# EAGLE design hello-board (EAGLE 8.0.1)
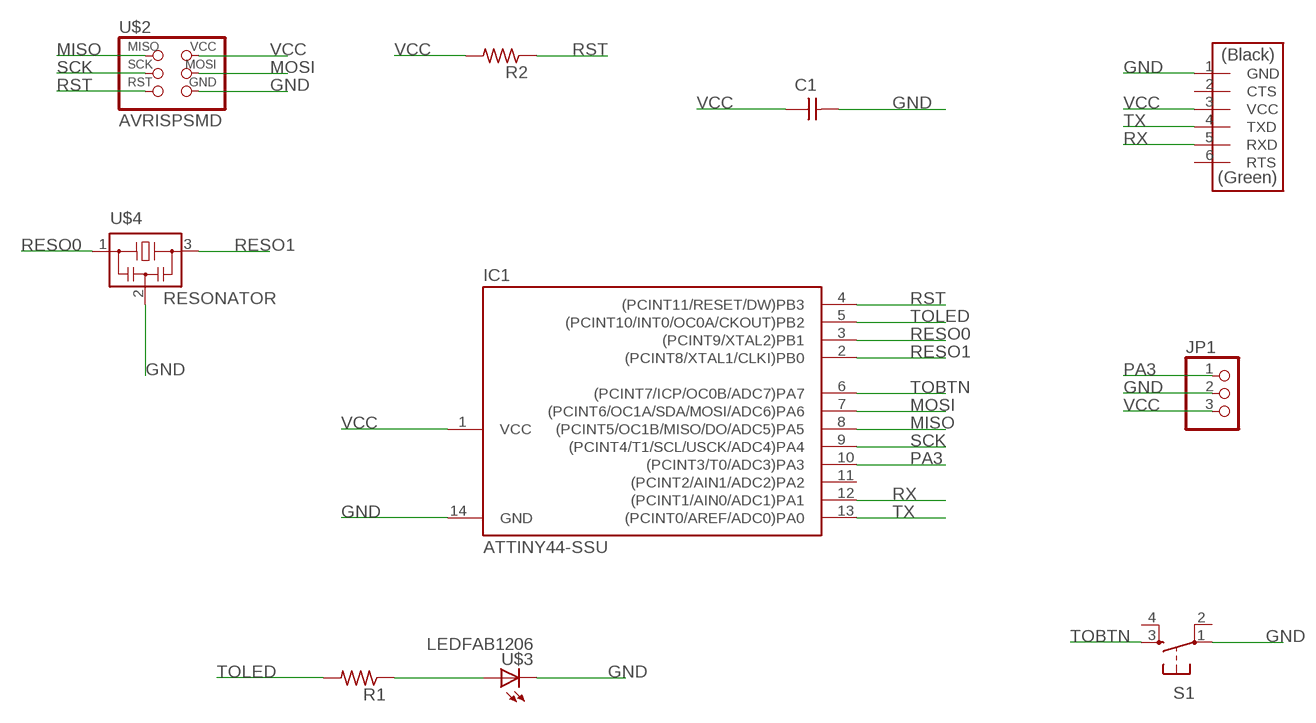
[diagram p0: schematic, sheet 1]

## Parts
C1  CAP-UNPOLARIZEDFAB  [C1206FAB]
IC1  ATTINY44-SSU  [SOIC14]
JP1  PINHD-1X3  [1X03]
R1  RES-US1206FAB  [R1206FAB]
R2  RES-US1206FAB  [R1206FAB]
S1  6MM_SWITCH6MM_SWITCH  [6MM_SWITCH]
U$1  FTDI-SMD-HEADER  [1X06SMD]
U$2  AVRISPSMD  [2X03SMD]
U$3  LEDFAB1206  [LED1206FAB]
U$4  RESONATOR  [EFOBM]

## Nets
GND: C1.2 IC1.14(GND) JP1.2 S1.1(P) U$1.1(GND) U$2.6(GND) U$3.2(C) U$4.2
MISO: IC1.8((PCINT5/OC1B/MISO/DO/ADC5)PA5) U$2.1(MISO)
MOSI: IC1.7((PCINT6/OC1A/SDA/MOSI/ADC6)PA6) U$2.4(MOSI)
N$12: R1.1 U$3.1(A)
PA3: IC1.10((PCINT3/T0/ADC3)PA3) JP1.1
RESO0: IC1.3((PCINT9/XTAL2)PB1) U$4.1
RESO1: IC1.2((PCINT8/XTAL1/CLKI)PB0) U$4.3
RST: IC1.4((PCINT11/RESET/DW)PB3) R2.1 U$2.5(RST)
RX: IC1.12((PCINT1/AIN0/ADC1)PA1) U$1.5(RXD)
SCK: IC1.9((PCINT4/T1/SCL/USCK/ADC4)PA4) U$2.3(SCK)
TOBTN: IC1.6((PCINT7/ICP/OC0B/ADC7)PA7) S1.3(S)
TOLED: IC1.5((PCINT10/INT0/OC0A/CKOUT)PB2) R1.2
TX: IC1.13((PCINT0/AREF/ADC0)PA0) U$1.4(TXD)
VCC: C1.1 IC1.1(VCC) JP1.3 R2.2 U$1.3(VCC) U$2.2(VCC)
Unconnected: IC1.11((PCINT2/AIN1/ADC2)PA2) S1.2(P1) S1.4(S1) U$1.2(CTS) U$1.6(RTS)

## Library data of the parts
C1 = 01fab:CAP-UNPOLARIZED
IC1 = 01fab:ATTINY44
JP1 = pinhead:PINHD-1X3: PIN HEADER
R1 R2 = 01fab:RES-US: Resistor (US Symbol)
S1 = 01fab:6MM_SWITCH: OMRON SWITCH
U$1 = 01fab:FTDI-SMD-HEADER
U$2 = 01fab:AVRISP
U$3 = 01fab:LED: LED
U$4 = 01fab:RESONATOR

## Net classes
0 default: width 0.406 mm, drill 0.406 mm, clearance 0.406 mm

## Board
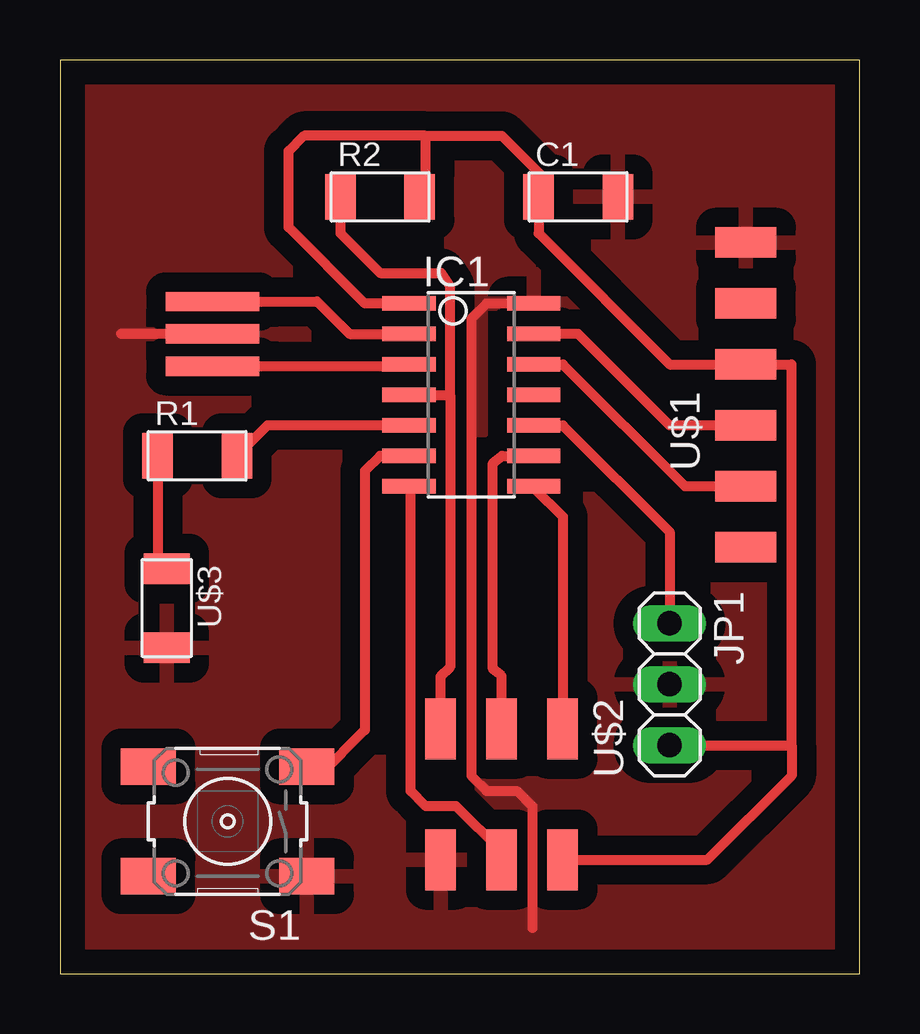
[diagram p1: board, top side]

Size 33.33 x 38.09 mm. Coordinates in mm from the lower left corner, seen from the top.
Outline: 0,0 33.33,0 33.33,38.09 0,38.09 0,0
Copper layers (1*16): Top 0.035mm / dielectric 1.5mm / Bottom 0.035mm
Design rules "default *": minimum track width 16mil, minimum drill 24mil, track to track 16mil, track to pad 16mil, pad to pad 16mil, via to via 16mil, smd to smd 16mil, copper to edge 40mil, drill to drill 8mil, minimum pad ring 10mil, minimum via ring 8mil, stop-mask expansion 4mil, vias tented up to drill 0mil, thermal gap 32mil

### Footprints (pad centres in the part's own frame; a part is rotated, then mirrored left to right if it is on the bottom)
C1206FAB = smd 1.27 x 1.905: 1 -1.651,0; 2 1.651,0
SOIC14 = smd 0.61 x 2.21: 1 -3.81,-2.603; 2 -2.54,-2.603; 3 -1.27,-2.603; 4 0,-2.603; 5 1.27,-2.603; 6 2.54,-2.603; 7 3.81,-2.603; 8 3.81,2.603; 9 2.54,2.603; 10 1.27,2.603; 11 0,2.603; 12 -1.27,2.603; 13 -2.54,2.603; 14 -3.81,2.603
1X03 = drill 1.016 long: 1 -2.54,0; 2 0,0; 3 2.54,0
R1206FAB = smd 1.27 x 1.905: 1 -1.651,0; 2 1.651,0
6MM_SWITCH = smd 2.286 x 1.524: 1 -3.302,2.286; 2 3.302,2.286; 3 -3.302,-2.286; 4 3.302,-2.286
1X06SMD = smd 2.54 x 1.27: 1 0,6.35; 2 0,3.81; 3 0,1.27; 4 0,-1.27; 5 0,-3.81; 6 0,-6.35
2X03SMD = smd 2.54 x 1.27: 1 -2.54,2.54; 2 2.92,2.54; 3 -2.54,0; 4 2.92,0; 5 -2.54,-2.54; 6 2.92,-2.54
LED1206FAB = smd 1.27 x 1.905: 1 -1.651,0; 2 1.651,0
EFOBM = smd 0.8 x 3.9: 1 -1.35,0; 2 0,0; 3 1.35,0

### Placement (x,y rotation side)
C1  21.59,32.38 0 top
IC1  17.14,24.13 270 top
JP1  25.4,12.06 270 top
R1  5.71,21.59 0 top
R2  13.34,32.38 0 top
S1  6.99,6.35 180 top
U$1  28.57,24.13 0 top
U$2  18.4,7.67 270 top
U$3  4.45,15.24 270 top
U$4  6.35,26.67 90 top

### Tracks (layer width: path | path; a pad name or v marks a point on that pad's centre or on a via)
GND
  Top 0.406: U$4.2 2.54,26.67 | 19.68,1.91 19.68,6.99 19.05,7.62 17.78,7.62 17.14,8.26 17.14,27.3 17.78,27.94 IC1.14
  pour Top (isolate 0.813): -0.64,39.37 34.29,39.37 34.29,-1.91 -0.64,-1.91
MISO
  Top 0.406: IC1.8 19.75,20.26 20.95,19.05 20.95,16.57 U$2.1
MOSI
  Top 0.406: U$2.4 18.4,5.09 16.51,6.99 15.24,6.99 14.61,7.62 14.61,20.26 IC1.7
N$12
  Top 0.406: R1.1 4.06,17.27 U$3.1
PA3
  Top 0.406: IC1.10 20.95,22.86 25.4,18.41 JP1.1
RESO0
  Top 0.406: U$4.1 14.46,25.32 IC1.3
RESO1
  Top 0.406: U$4.3 10.71,28.02 12.06,26.67 IC1.2
RST
  Top 0.406: R2.1 11.68,30.86 13.34,29.21 15.88,29.21 16.26,28.65 16.26,24.13 | 16.26,24.13 16.26,12.78 15.86,12.38 U$2.5 15.88,10.22 | IC1.4 16.26,24.13
RX
  Top 0.406: IC1.12 20.95,25.4 26.04,20.32 U$1.5
SCK
  Top 0.406: U$2.3 18.4,12.41 18.03,12.7 18.03,21.29 18.41,21.59 IC1.9
TOBTN
  Top 0.406: IC1.6 13.34,21.59 12.7,20.95 12.7,10.16 10.79,8.26 10.54,8.26 S1.3
TOLED
  Top 0.406: R1.2 8.64,22.86 IC1.5
TX
  Top 0.406: U$1.4 25.4,22.86 21.59,26.67 IC1.13
VCC
  Top 0.406: 30.48,9.53 30.48,25.4 U$1.3 25.4,25.4 19.94,30.86 C1.1 20.32,32.77 20.32,33.02 18.41,34.92 15.24,34.92 | 30.48,9.53 30.48,8.26 26.98,4.75 U$2.2 | IC1.1 12.7,27.94 9.53,31.11 9.53,34.29 10.16,34.92 15.24,34.92 | R2.2 15.24,32.38 15.24,34.92 | JP1.3 30.48,9.53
